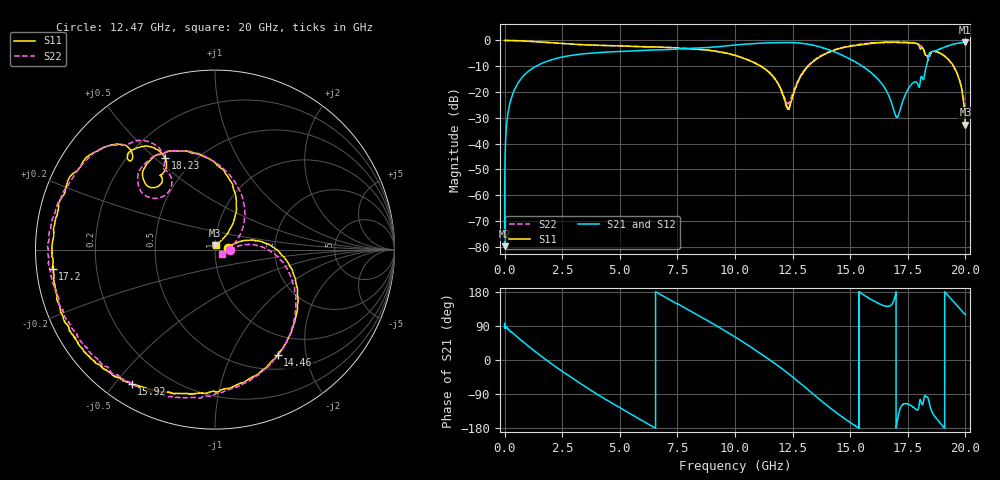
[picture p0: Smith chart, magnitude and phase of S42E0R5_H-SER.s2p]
!{S42E0R5}
!Johanson Technology Inc.
!www.johansontechnology.com
!Test Board Conditions:
!Substrate Type  RO4350B
!Substrate Thickness  50 mil
!Substrate Dk  3.66
!TL Type: GCPW
!TL Trace Width  60 mil
!TL Gap  10 mil
!Electrode orientation  Horizontal
!DUT TOPOLOGY	SERIES
!Mounting Pad LxW  14x55 mil
! Created Wed Nov 25 21:24:17 2020
# khz S ma R 50
! 2 Port Network Data from SP1.SP block
! freq  magS11  angS11  magS21  angS21  magS12  angS12  magS22  angS22
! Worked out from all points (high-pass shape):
!   20001 points, 300 kHz to 20 GHz, reference 50 ohm
!   highest |S21| = -0.71 dB at 19.99 GHz (marker M1); lowest = -79.7 dB at 300 kHz (marker M2)
!   |S21| within 3 dB of the highest: 6.449 GHz to 14.11 GHz (7.661 GHz wide, 74.5 % of centre); 18.79 GHz to end of sweep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
!   lowest |S11| = -32.6 dB at 20 GHz (marker M3), VSWR 1.05, Z = 50.1 + j2.35 ohm
!   |S11| at or under -10 dB: 11.13 GHz to 13.17 GHz (2.04 GHz wide, 16.8 % of centre); 13.17057 GHz to 13.17161 GHz (1.041 MHz wide, 0.0079 % of centre); 19.49 GHz to end of sweep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
!   |S22| runs from -27.2 to 0.0 dB; largest |S21 - S12| = 0.012
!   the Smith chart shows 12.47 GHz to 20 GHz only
!   S11 on the Smith chart (normalised r, x): 12.47 GHz: 1.16, +0.02; 14.46 GHz: 0.69, -1.53; 15.92 GHz: 0.08, -0.55; 17.2 GHz: 0.05, -0.06; 18.23 GHz: 0.35, +0.54; 20 GHz: 1.00, +0.05
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300  0.997 -0.2  0.0001031 96.9  1.908e-05 63.8  0.9966 -0.1
135300  0.9993 -7.1  0.03553 82.6  0.03579 82.4  0.9978 -7.1
513300  0.9909 -27.1  0.1326 62.9  0.1331 62.9  0.9908 -27.2
1767300  0.9214 -87.9  0.3824 2.0  0.3838 1.9  0.9198 -88.1
3334300  0.8303 -154.9  0.5457 -63.7  0.5452 -63.8  0.829 -152.2
4680300  0.7904 155.6  0.6028 -114.5  0.6022 -114.6  0.7909 156.0
6667300  0.7441 88.4  0.6579 176.1  0.656 175.9  0.7453 84.6
8473300  0.6698 25.6  0.7162 115.3  0.7134 115.3  0.6705 25.1
1.00003e7  0.5149 -26.8  0.8161 61.0  0.8163 61.2  0.5136 -28.8
1.13703e7  0.267 -71.3  0.8943 6.0  0.8973 6.2  0.2646 -78.9
1.22703e7  0.04939 -48.0  0.912 -33.7  0.9136 -33.9  0.06074 -48.6
1.24723e7  0.07326 8.2  0.9062 -43.3  0.9085 -43.5  0.08404 -1.5
1.33343e7  0.3694 -4.1  0.8165 -86.9  0.8193 -86.7  0.3789 -10.0
1.44593e7  0.684 -59.3  0.5647 -141.7  0.5705 -141.9  0.6919 -60.4
1.59183e7  0.8825 -121.8  0.2351 159.3  0.236 159.1  0.8814 -123.2
1.66673e7  0.9238 -148.7  0.08727 141.8  0.08524 143.1  0.9154 -156.6
1.71993e7  0.9113 -173.2  0.05085 -124.1  0.05038 -122.7  0.9309 -179.6
1.82283e7  0.5791 118.6  0.2142 -94.5  0.2171 -94.8  0.5808 119.1
1.84933e7  0.5653 135.2  0.6008 -127.8  0.6039 -127.5  0.557 140.1
1.94523e7  0.334 70.4  0.837 156.1  0.8355 155.9  0.3252 61.7
1.99913e7  0.02747 77.8  0.9213 120.0  0.9131 119.9  0.04619 -27.5
2e7  0.0235 85.8  0.9203 119.3  0.9147 119.4  0.04351 -33.5
